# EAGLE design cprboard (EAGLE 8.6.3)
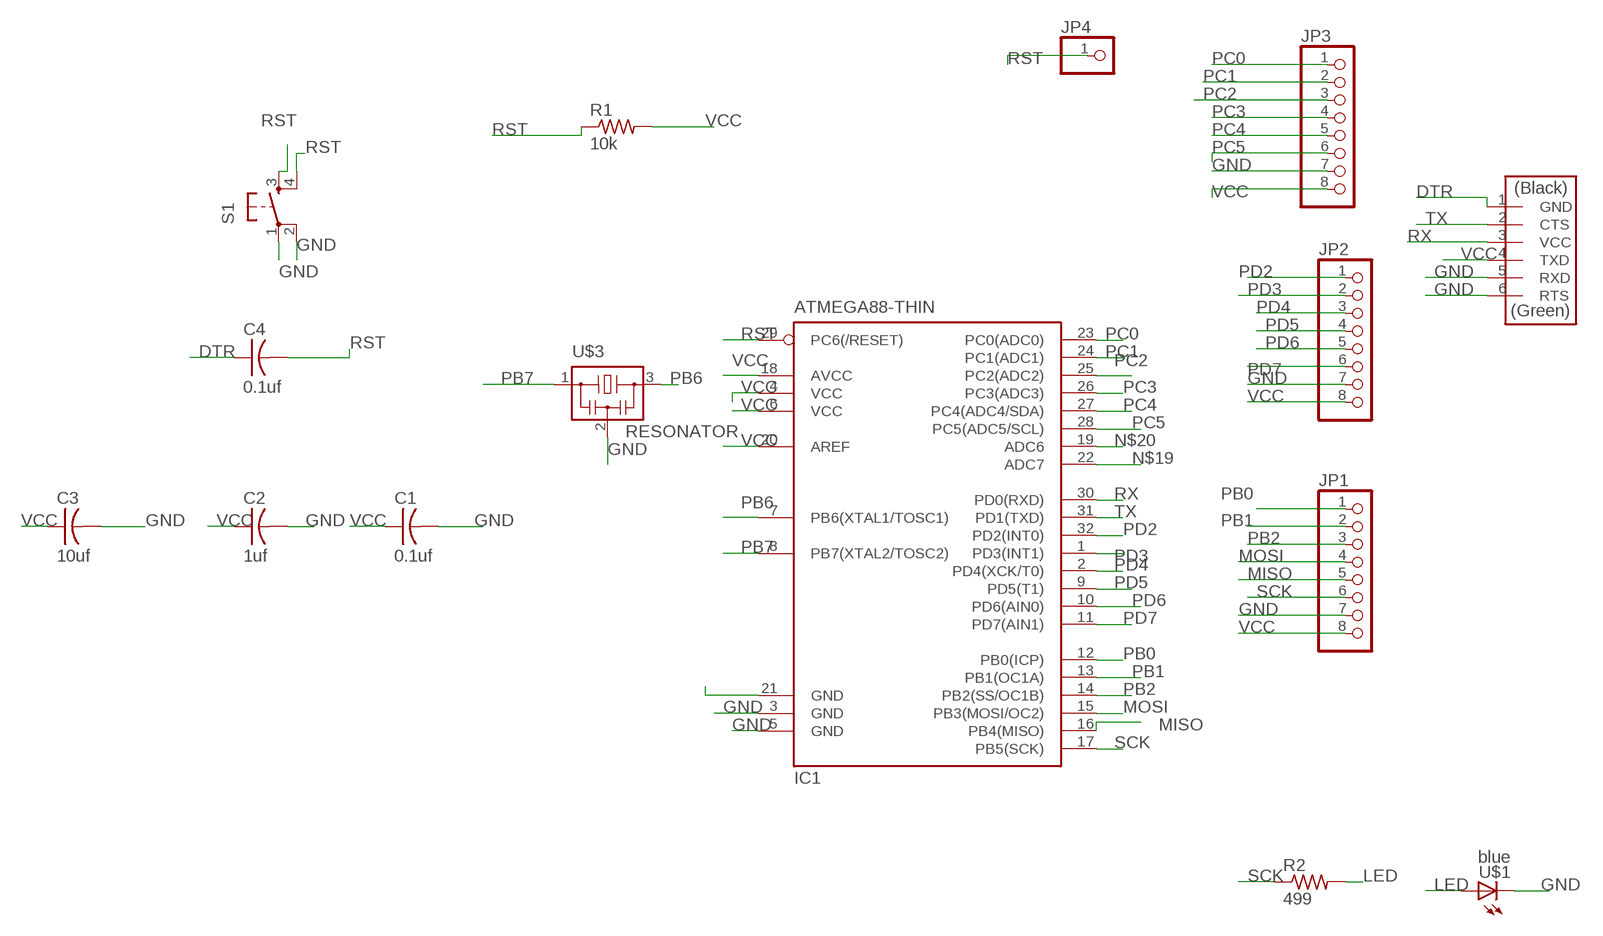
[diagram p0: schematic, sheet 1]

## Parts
C1  0.1uf  CAP-US1206K  [C1206K]
C2  1uf  CAP-US1206K  [C1206K]
C3  10uf  CAP-US1206K  [C1206K]
C4  0.1uf  CAP-US1206K  [C1206K]
IC1  ATMEGA88-THIN  [TQFP32-08THIN]
JP1  PINHD-1X8  [1X08]
JP2  PINHD-1X8  [1X08]
JP3  PINHD-1X8  [1X08]
JP4  PINHD-1X1  [1X01]
R1  10k  RES-US1206  [R1206]
R2  499  RES-US1206  [R1206]
S1  6MM_SWITCH6MM_SWITCH  [6MM_SWITCH]
U$1  blue  LED  [LED1206]
U$3  RESONATOR  [EFOBM]
U$4  FTDI-SMD-HEADER  [1X06SMD]

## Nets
DTR: C4.1 U$4.1(GND)
GND: C1.2 C2.2 C3.2 IC1.3(GND) IC1.5(GND) IC1.21(GND) JP1.7 JP2.7 JP3.7 S1.1(P) S1.2(P1) U$1.2(C) U$3.2 U$4.5(RXD) U$4.6(RTS)
LED: R2.2 U$1.1(A)
MISO: IC1.16(PB4(MISO)) JP1.5
MOSI: IC1.15(PB3(MOSI/OC2)) JP1.4
N$19: IC1.22(ADC7)
N$20: IC1.19(ADC6)
PB0: IC1.12(PB0(ICP)) JP1.1
PB1: IC1.13(PB1(OC1A)) JP1.2
PB2: IC1.14(PB2(SS/OC1B)) JP1.3
PB6: IC1.7(PB6(XTAL1/TOSC1)) U$3.3
PB7: IC1.8(PB7(XTAL2/TOSC2)) U$3.1
PC0: IC1.23(PC0(ADC0)) JP3.1
PC1: IC1.24(PC1(ADC1)) JP3.2
PC2: IC1.25(PC2(ADC2)) JP3.3
PC3: IC1.26(PC3(ADC3)) JP3.4
PC4: IC1.27(PC4(ADC4/SDA)) JP3.5
PC5: IC1.28(PC5(ADC5/SCL)) JP3.6
PD2: IC1.32(PD2(INT0)) JP2.1
PD3: IC1.1(PD3(INT1)) JP2.2
PD4: IC1.2(PD4(XCK/T0)) JP2.3
PD5: IC1.9(PD5(T1)) JP2.4
PD6: IC1.10(PD6(AIN0)) JP2.5
PD7: IC1.11(PD7(AIN1)) JP2.6
RST: C4.2 IC1.29(PC6(/RESET)) JP4.1 R1.1 S1.3(S) S1.4(S1)
RX: IC1.30(PD0(RXD)) U$4.3(VCC)
SCK: IC1.17(PB5(SCK)) JP1.6 R2.1
TX: IC1.31(PD1(TXD)) U$4.2(CTS)
VCC: C1.1 C2.1 C3.1 IC1.4(VCC) IC1.6(VCC) IC1.18(AVCC) IC1.20(AREF) JP1.8 JP2.8 JP3.8 R1.2 U$4.4(TXD)

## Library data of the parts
C1-C4 = fab:CAP-US
IC1 = fab:ATMEGA88-THIN
JP1-JP3 = pinhead:PINHD-1X8: PIN HEADER
JP4 = pinhead:PINHD-1X1: PIN HEADER
R1 R2 = fab:RES-US: Resistor (US Symbol)
S1 = fab:6MM_SWITCH: OMRON SWITCH
U$1 = fab:LED: LED
U$3 = fab:RESONATOR
U$4 = fab:FTDI-SMD-HEADER

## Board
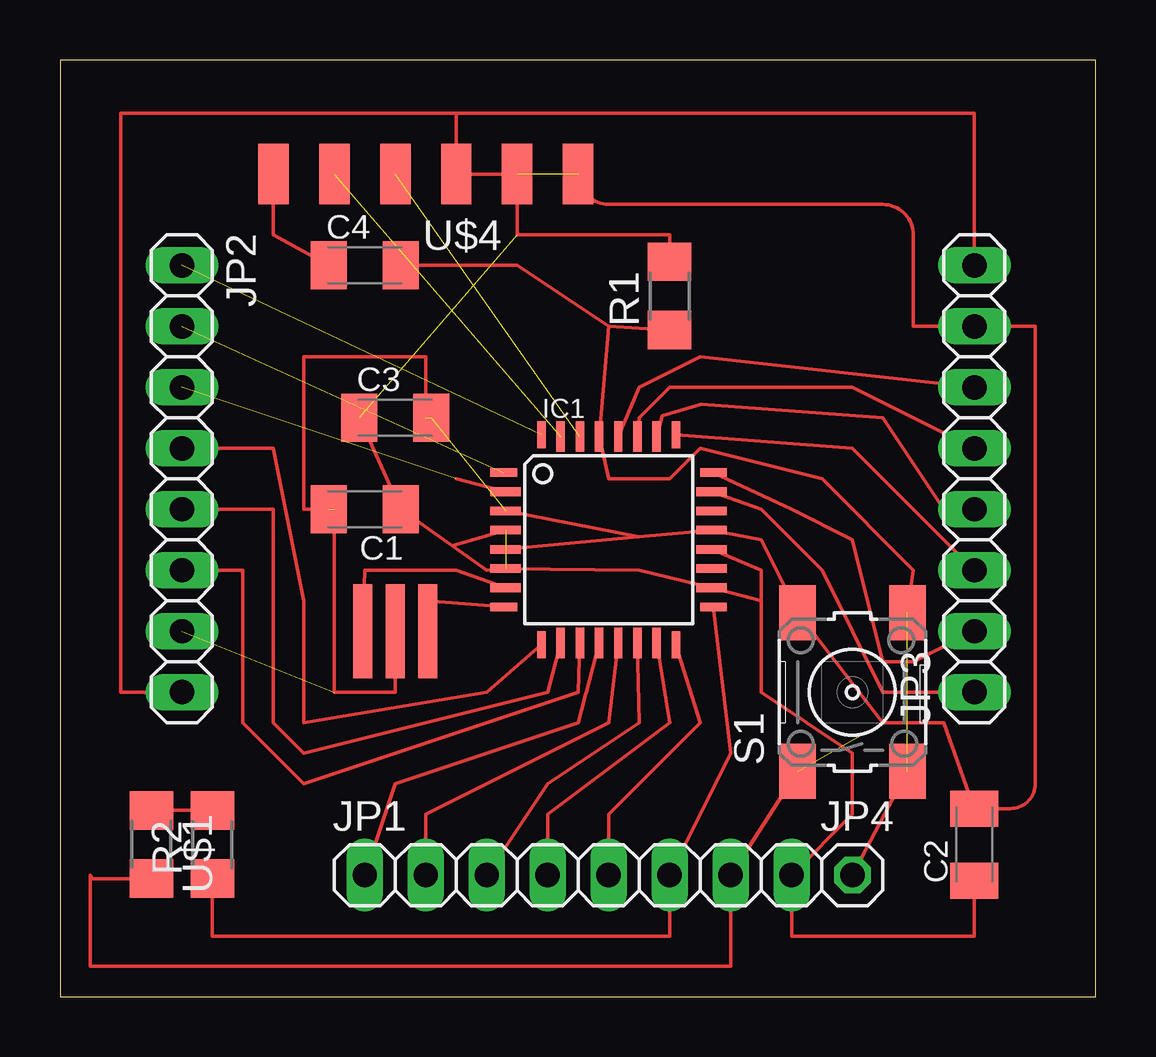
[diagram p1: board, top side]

Size 43.16 x 39.04 mm. Coordinates in mm from the lower left corner, seen from the top.
Outline: 0,0 43.16,0 43.16,39.04 0,39.04 0,0
Copper layers (1*16): Top 0.035mm / dielectric 1.5mm / Bottom 0.035mm
Design rules "default": minimum track width 6mil, minimum drill 0.35mm, track to track 6mil, track to pad 6mil, pad to pad 6mil, via to via 6mil, smd to smd 6mil, copper to edge 40mil, drill to drill 6mil, minimum pad ring 10mil, minimum via ring 8mil, stop-mask expansion 4mil, vias tented up to drill 0mil, thermal gap 10mil

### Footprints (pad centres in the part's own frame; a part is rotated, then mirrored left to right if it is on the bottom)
C1206K = smd 1.5 x 2: 1 -1.5,0; 2 1.5,0
TQFP32-08THIN = smd 1.118 x 0.356: 1 -4.369,2.8; 8 -4.369,-2.8; 17 4.369,-2.8; 24 4.369,2.8 | smd 1.27 x 0.356: 2 -4.293,2; 3 -4.293,1.2; 4 -4.293,0.4; 5 -4.293,-0.4; 6 -4.293,-1.2; 7 -4.293,-2; 18 4.293,-2; 19 4.293,-1.2; 20 4.293,-0.4; 21 4.293,0.4; 22 4.293,1.2; 23 4.293,2 | smd 0.356 x 1.118: 9 -2.8,-4.369; 16 2.8,-4.369; 25 2.8,4.369; 32 -2.8,4.369 | smd 0.356 x 1.27: 10 -2,-4.293; 14 1.2,-4.293; 15 2,-4.293; 26 2,4.293; 27 1.2,4.293; 31 -2,4.293 | smd 0.35 x 1.27: 11 -1.2,-4.293; 12 -0.4,-4.293; 13 0.4,-4.293; 28 0.4,4.293; 29 -0.4,4.293; 30 -1.2,4.293
1X08 = drill 1.016 long: 1 -8.89,0; 2 -6.35,0; 3 -3.81,0; 4 -1.27,0; 5 1.27,0; 6 3.81,0; 7 6.35,0; 8 8.89,0
1X01 = drill 1.016 octagon: 1 0,0
R1206 = smd 1.6 x 1.803: 1 -1.422,0; 2 1.422,0
6MM_SWITCH = smd 2.286 x 1.524: 1 -3.302,2.286; 2 3.302,2.286; 3 -3.302,-2.286; 4 3.302,-2.286
LED1206 = smd 1.6 x 1.803: 1 -1.422,0; 2 1.422,0
EFOBM = smd 0.8 x 3.9: 1 -1.35,0; 2 0,0; 3 1.35,0
1X06SMD = smd 2.54 x 1.27: 1 0,6.35; 2 0,3.81; 3 0,1.27; 4 0,-1.27; 5 0,-3.81; 6 0,-6.35

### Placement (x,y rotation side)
C1  12.7,20.32 180 top
C2  38.1,6.35 90 top
C3  13.97,24.13 0 top
C4  12.7,30.48 0 top
IC1  22.86,19.05 0 top
JP1  21.59,5.08 0 top
JP2  5.08,21.59 270 top
JP3  38.1,21.59 90 top
JP4  33.02,5.08 0 top
R1  25.4,29.21 90 top
R2  6.35,6.35 90 top
S1  33.02,12.7 90 top
U$1  3.81,6.35 270 top
U$3  13.97,15.24 180 top
U$4  15.24,34.29 90 top

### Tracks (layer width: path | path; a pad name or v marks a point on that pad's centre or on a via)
DTR
  Top 0.152: U$4.1 8.89,31.75 C4.1
GND  (6 unrouted)
  Top 0.152: U$3.2 13.97,12.7 11.43,12.7 11.43,20.32 10.16,20.32 10.16,26.67 15.24,26.67 15.24,24.13 | S1.1 JP1.7 27.94,1.27 1.27,1.27 1.27,5.08 arc90 1.42,4.93 U$1.2 | IC1.5 24.12,19.17 | 24.12,19.17 IC1.21 29.21,19.05 S1.2 34.29,11.43 36.83,11.43 C2.2 39.6,7.85 arc90 40.64,8.89 40.64,27.94 JP3.7 35.56,27.94 35.56,31.75 arc90 34.29,33.02 22.86,33.02 arc-90 U$4.6 | IC1.3 24.12,19.17
LED
  Top 0.152: R2.2 U$1.1
MISO
  Top 0.152: JP1.5 22.86,7.62 26.67,11.43 IC1.16
MOSI
  Top 0.152: JP1.4 20.32,7.62 25.4,11.43 IC1.15
PB0
  Top 0.152: JP1.1 13.97,8.89 21.59,11.43 21.89,12.56 21.89,12.57 21.92,12.68 IC1.12
PB1
  Top 0.152: IC1.13 22.86,11.43 15.24,7.62 JP1.2
PB2
  Top 0.152: JP1.3 20.32,8.89 24.13,11.43 IC1.14
PB6
  Top 0.152: U$3.3 12.7,17.78 16.51,17.78 IC1.7
PB7
  Top 0.152: U$3.1 15.24,16.51 IC1.8
PC0
  Top 0.152: JP3.1 34.29,12.7 31.75,17.78 29.21,20.32 IC1.23
PC1
  Top 0.152: JP3.2 35.56,13.97 34.29,13.97 33.02,19.05 30.48,20.32 IC1.24
PC2
  Top 0.152: IC1.25 33.02,22.86 JP3.3
PC3
  Top 0.152: IC1.26 25.09,24.21 26.51,24.64 26.71,24.7 34.29,24.13 | 34.29,24.13 36.83,20.32 JP3.4 | 34.29,24.13
PC4
  Top 0.152: IC1.27 24.13,24.13 25.4,25.4 33.02,25.4 JP3.5
PC5
  Top 0.152: IC1.28 24.13,25.4 26.67,26.67 JP3.6
PD2  (1 unrouted)
PD3  (1 unrouted)
PD4  (1 unrouted)
  Top 0.152: IC1.2 16.51,21.59 | 16.51,21.59
PD5
  Top 0.152: IC1.9 17.78,12.7 10.16,11.43 10.16,16.51 8.89,22.86 JP2.4
PD6
  Top 0.152: JP2.5 8.89,20.32 8.89,11.43 10.16,10.16 20.32,12.7 IC1.10
PD7
  Top 0.152: JP2.6 7.62,17.78 7.62,11.43 10.16,8.89 21.59,12.7 IC1.11
RST  (1 unrouted)
  Top 0.152: S1.3 JP4.1 | 22.86,27.94 IC1.29 22.86,21.59 25.4,21.59 26.67,22.86 31.75,21.59 35.56,17.78 S1.4 | 22.86,27.94 R1.1 | 22.86,27.94 19.05,30.48 C4.2
RX  (1 unrouted)
SCK
  Top 0.152: IC1.17 27.94,10.16 JP1.6 25.4,2.54 6.35,2.54 R2.1
TX  (1 unrouted)
VCC  (2 unrouted)
  Top 0.152: C3.1 12.99,22.99 13.68,21.46 C1.1 17.78,17.78 IC1.6 24.13,17.78 IC1.18 29.21,16.51 | C2.1 38.1,2.54 30.48,2.54 JP1.8 33.02,7.62 33.02,10.16 29.21,12.7 29.21,16.51 | IC1.20 29.21,17.78 29.21,16.51 | IC1.4 16.34,18.8 | R1.2 25.4,31.75 19.05,31.75 19.05,34.29 U$4.4 16.51,36.83 | 16.51,36.83 38.1,36.83 JP3.8 | 16.51,36.83 2.54,36.83 2.54,12.7 JP2.8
